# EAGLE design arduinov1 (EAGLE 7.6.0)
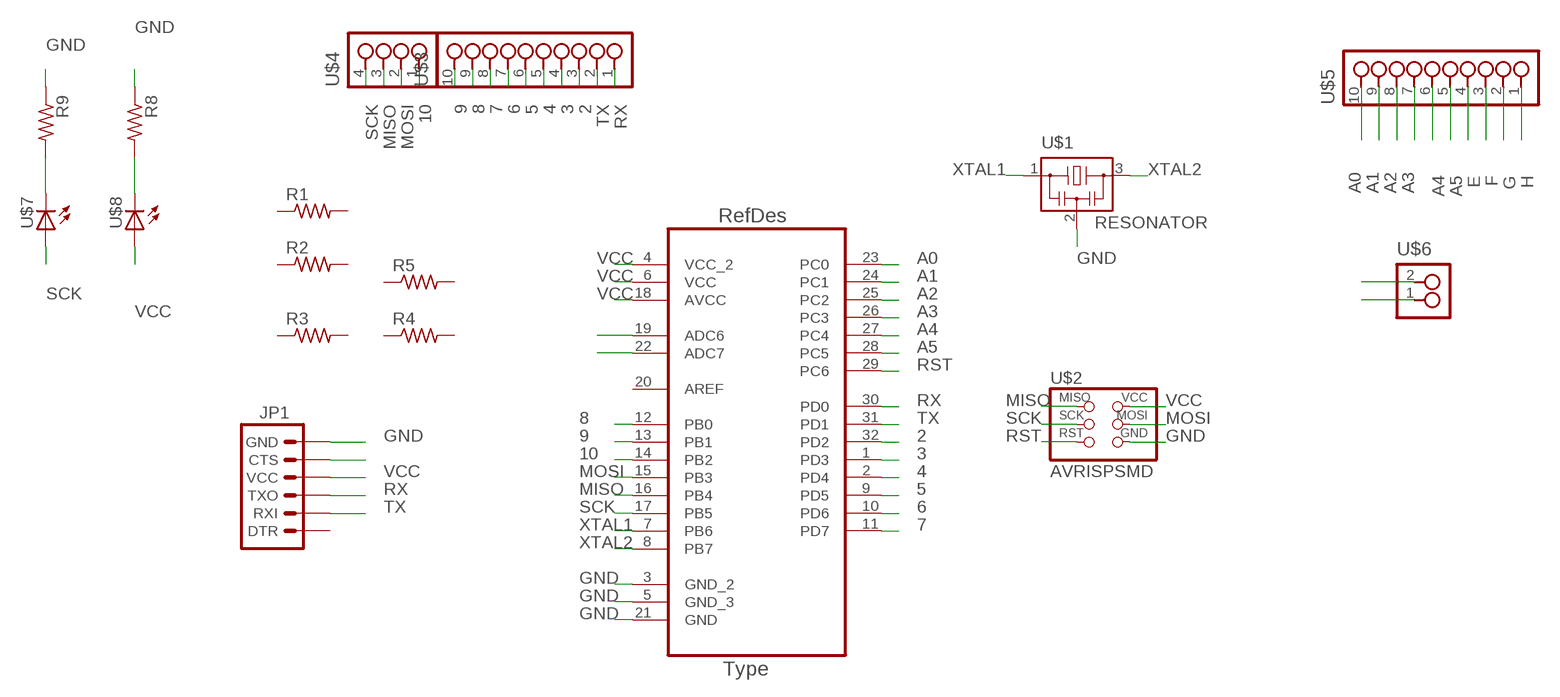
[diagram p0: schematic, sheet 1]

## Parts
JP1  ARDUINO_SERIAL_PROGRAMSMD  [1X06-SMD]
R1  RES-US1206FAB  [R1206FAB]
R2  RES-US1206FAB  [R1206FAB]
R3  RES-US1206FAB  [R1206FAB]
R4  RES-US1206FAB  [R1206FAB]
R5  RES-US1206FAB  [R1206FAB]
R8  RES-US1206FAB  [R1206FAB]
R9  RES-US1206FAB  [R1206FAB]
U1  ATMEGA328P-AU  [QFP80P900X900X120-32N]
U$1  RESONATOR  [EFOBM]
U$2  AVRISPSMD  [2X03SMD]
U$3  10_PIN_HEADERHEADER  [SMT_PINS_10]
U$4  4_PIN_HEADERHEADER  [SMT_PINS_4]
U$5  10_PIN_HEADERHEADER  [SMT_PINS_10]
U$6  2_PIN_HEADERHEADER  [SMT_PINS_2]
U$7  LED1206  [1206]
U$8  LED1206  [1206]

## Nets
2: U1.32(PD2) U$3.3
3: U1.1(PD3) U$3.4
4: U1.2(PD4) U$3.5
5: U1.9(PD5) U$3.6
6: U1.10(PD6) U$3.7
7: U1.11(PD7) U$3.8
8: U1.12(PB0) U$3.9
9: U1.13(PB1) U$3.10
10: U1.14(PB2) U$4.1
A0: U1.23(PC0) U$5.10
A1: U1.24(PC1) U$5.9
A2: U1.25(PC2) U$5.8
A3: U1.26(PC3) U$5.7
A4: U1.27(PC4) U$5.6
A5: U1.28(PC5) U$5.5
A6: U1.19(ADC6) U$6.1
A7: U1.22(ADC7) U$6.2
E: U$5.4
F: U$5.3
G: U$5.2
GND: JP1.6(GND) R8.1 R9.1 U1.3(GND_2) U1.5(GND_3) U1.21(GND) U$1.2 U$2.6(GND)
H: U$5.1
MISO: U1.16(PB4) U$2.1(MISO) U$4.3
MOSI: U1.15(PB3) U$2.4(MOSI) U$4.2
N$4: JP1.5(CTS)
N$7: R9.2 U$7.2(C)
N$8: R8.2 U$8.2(C)
RST: U1.29(PC6) U$2.5(RST)
RX: JP1.3(TXO) U1.30(PD0) U$3.1
SCK: U1.17(PB5) U$2.3(SCK) U$4.4 U$7.1(A)
TX: JP1.2(RXI) U1.31(PD1) U$3.2
VCC: JP1.4(VCC) U1.4(VCC_2) U1.6(VCC) U1.18(AVCC) U$2.2(VCC) U$8.1(A)
XTAL1: U1.7(PB6) U$1.1
XTAL2: U1.8(PB7) U$1.3
Unconnected: JP1.1(DTR) R1.1 R1.2 R2.1 R2.2 R3.1 R3.2 R4.1 R4.2 R5.1 R5.2 U1.20(AREF)

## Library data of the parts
JP1 = SparkFun-Connectors:ARDUINO_SERIAL_PROGRAM: FTDI connector footprints
R1-R5 R8 R9 = fab:RES-US: Resistor (US Symbol)
U1 = Atmel-ATMEGA328P-AU:ATMEGA328P-AU; DESCRIPTION: 8-bit Microcontroller with In-System Programmable Flash; MPN: ATMEGA328P-AU; OC_FARNELL: 1715486; OC_NEWARK: 14R4631; PACKAGE: TQFP-32; SUPPLIER: Atmel
U$1 = fab:RESONATOR
U$2 = fab:AVRISP
U$3 U$5 = FabLab:10_PIN_HEADER
U$4 = FabLab:4_PIN_HEADER: 4 SMT pin pads
U$6 = FabLab:2_PIN_HEADER: 2 SMT pin pads
U$7 U$8 = FabLab:LED

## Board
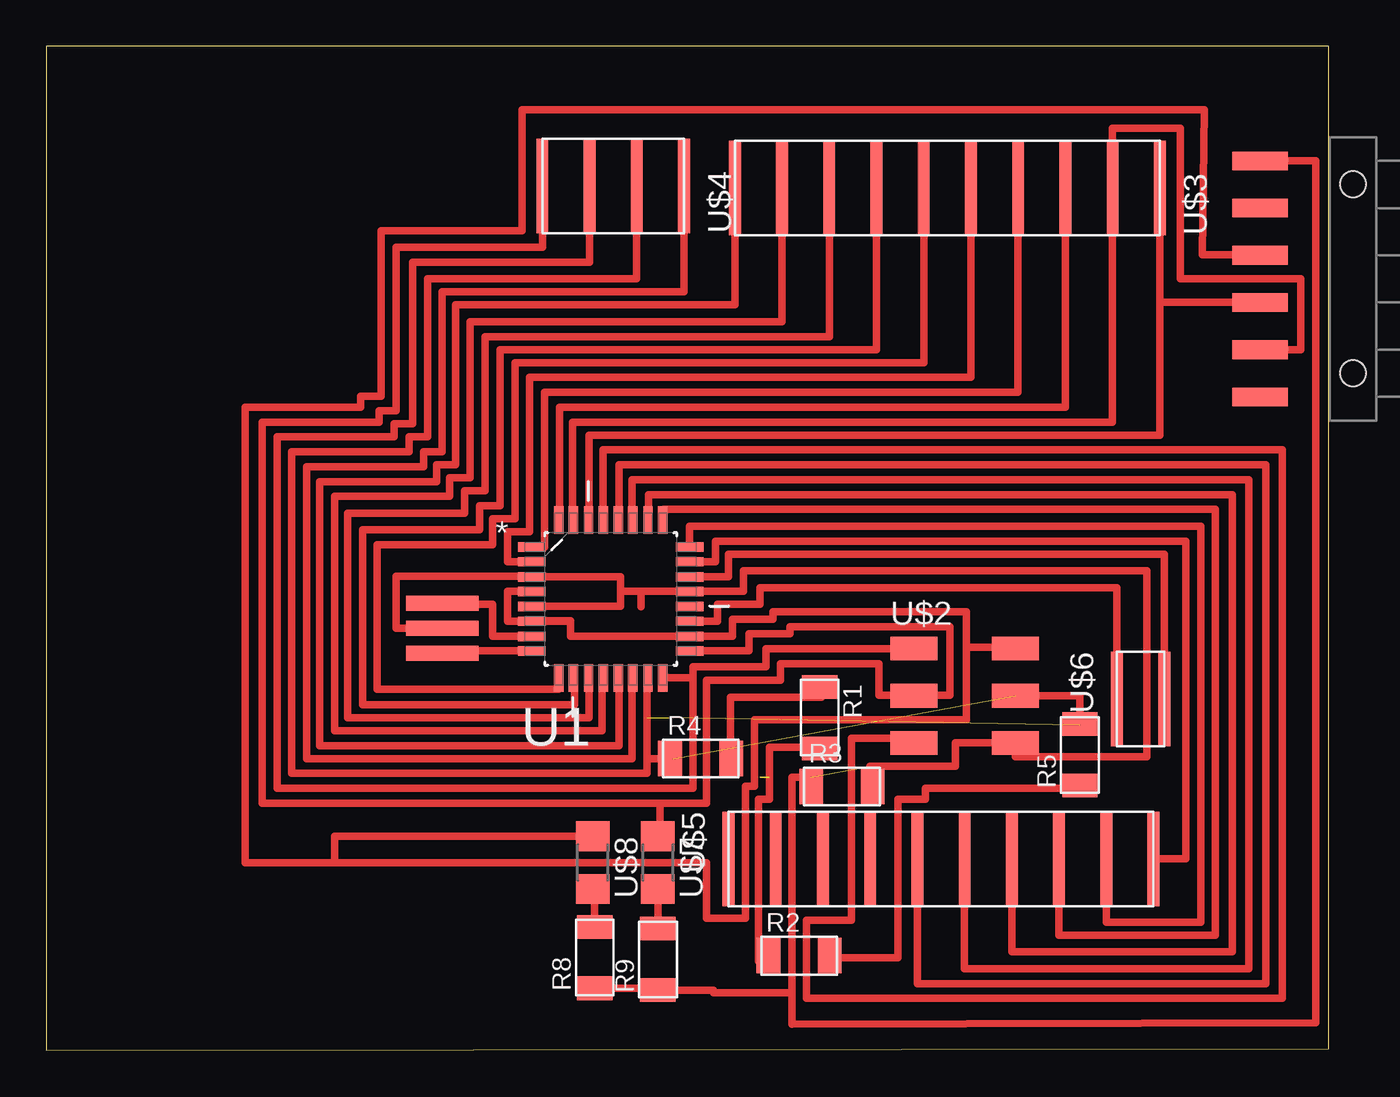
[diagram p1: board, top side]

Size 69 x 54 mm. Coordinates in mm from the lower left corner, seen from the top.
Outline: 0,0 69,0.1 69,54 0,54 0,0
Copper layers (1*16): Top 0.035mm / dielectric 1.5mm / Bottom 0.035mm
Design rules "default": minimum track width 10mil, minimum drill 24mil, track to track 8mil, track to pad 8mil, pad to pad 8mil, via to via 8mil, smd to smd 8mil, copper to edge 40mil, drill to drill 8mil, minimum pad ring 10mil, minimum via ring 8mil, stop-mask expansion 4mil, vias tented up to drill 0mil, thermal gap 10mil

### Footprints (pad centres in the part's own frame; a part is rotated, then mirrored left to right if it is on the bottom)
1X06-SMD = smd 1 x 3: 1 -6.35,5; 2 -3.81,5; 3 -1.27,5; 4 1.27,5; 5 3.81,5; 6 6.35,5 | hole 1.4: -5.08,0; 5.08,0
R1206FAB = smd 1.27 x 1.905: 1 -1.651,0; 2 1.651,0
QFP80P900X900X120-32N = smd 1.473 x 0.508: 1 -4.242,2.794; 2 -4.242,2.007; 3 -4.242,1.194; 4 -4.242,0.406; 5 -4.242,-0.406; 6 -4.242,-1.194; 7 -4.242,-2.007; 8 -4.242,-2.794; 17 4.242,-2.794; 18 4.242,-2.007; 19 4.242,-1.194; 20 4.242,-0.406; 21 4.242,0.406; 22 4.242,1.194; 23 4.242,2.007; 24 4.242,2.794 | smd 0.508 x 1.473: 9 -2.794,-4.242; 10 -2.007,-4.242; 11 -1.194,-4.242; 12 -0.406,-4.242; 13 0.406,-4.242; 14 1.194,-4.242; 15 2.007,-4.242; 16 2.794,-4.242; 25 2.794,4.242; 26 2.007,4.242; 27 1.194,4.242; 28 0.406,4.242; 29 -0.406,4.242; 30 -1.194,4.242; 31 -2.007,4.242; 32 -2.794,4.242
EFOBM = smd 0.8 x 3.9: 1 -1.35,0; 2 0,0; 3 1.35,0
2X03SMD = smd 2.54 x 1.27: 1 -2.54,2.54; 2 2.92,2.54; 3 -2.54,0; 4 2.92,0; 5 -2.54,-2.54; 6 2.92,-2.54
SMT_PINS_10 = smd 5.08 x 0.635: 1 0,0; 2 0,2.54; 3 0,5.08; 4 0,7.62; 5 0,10.16; 6 0,12.7; 7 0,15.24; 8 0,17.78; 9 0,20.32; 10 0,22.86
SMT_PINS_4 = smd 5.08 x 0.635: 1 0,0; 2 0,2.54; 3 0,5.08; 4 0,7.62
SMT_PINS_2 = smd 5.08 x 0.635: 1 0,0; 2 0,2.54
1206 = smd 1.6 x 1.803: 1 -1.422,0; 2 1.422,0

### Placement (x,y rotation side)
JP1  70.3,41.5 90 top
R1  41.6,17.9 270 top
R2  40.5,5.1 0 top
R3  42.8,14.2 0 top
R4  35.2,15.7 0 top
R5  55.6,15.9 90 top
R8  29.5,5 90 top
R9  32.9,4.9 90 top
U1  30.36,24.28 0 top
U$1  21.3,22.71 270 top
U$2  49.22,19.08 0 top
U$3  59.9,46.4 90 top
U$4  34.3,46.5 90 top
U$5  36.7,10.3 270 top
U$6  57.6,18.9 270 top
U$7  32.9,10.1 270 top
U$8  29.4,10.1 270 top

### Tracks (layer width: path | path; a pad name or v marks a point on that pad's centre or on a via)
2
  Top 0.406: U1.32 27.6,28.52 27.6,34.6 54.82,34.6 U$3.3
3
  Top 0.406: U1.1 26.8,27.07 26.8,35.4 52.28,35.4 U$3.4
4
  Top 0.406: U1.2 24.8,26.29 24.8,27.9 26,27.9 26,36.2 49.74,36.2 U$3.5
5
  Top 0.406: U$3.6 47.2,37 25.2,37 25.2,28.6 24,28.6 24,27.2 17.8,27.2 17.8,19.44 27.57,19.44 U1.9
6
  Top 0.406: U1.10 28.4,20.04 28.4,18.6 17,18.6 17,28 23.3,28 23.3,29.3 24.4,29.3 24.4,37.7 44.66,37.7 U$3.7
7
  Top 0.406: U1.11 29.2,20.04 29.2,17.9 16.2,17.9 16.2,28.9 22.5,28.9 22.5,30.1 23.6,30.1 23.6,38.4 42.12,38.4 U$3.8
8
  Top 0.406: U1.12 29.9,20.04 29.9,17.2 15.5,17.2 15.5,29.8 21.7,29.8 21.7,30.8 22.8,30.8 22.8,39.2 39.58,39.2 U$3.9
9
  Top 0.406: U1.13 30.8,20.04 30.8,16.4 14.7,16.4 14.7,30.6 21,30.6 21,31.5 22,31.5 22,40.1 37.04,40.1 U$3.10
10
  Top 0.406: U1.14 31.5,20.04 31.5,15.7 14,15.7 14,31.4 20.3,31.4 20.3,32.2 21.3,32.2 21.3,40.8 34.3,40.8 U$4.1
A0
  Top 0.406: U1.23 36,26.29 36,27.4 61.3,27.4 61.3,10.3 U$5.10
A1
  Top 0.406: U1.24 34.6,28.2 62.1,28.2 62.1,6.9 57.02,6.9 U$5.9
A2
  Top 0.406: U$5.8 54.48,6.2 62.9,6.2 62.9,29.1 33.2,29.1 33.2,28.52 U1.25
A3
  Top 0.406: U1.26 32.4,28.52 32.4,29.9 63.8,29.9 63.8,5.3 51.94,5.3 U$5.7
A4
  Top 0.406: U1.27 31.5,28.52 31.5,30.7 64.7,30.7 64.7,4.4 49.4,4.4 U$5.6
A5
  Top 0.406: U1.28 30.8,28.52 30.8,31.5 65.6,31.5 65.6,3.6 46.86,3.6 U$5.5
A6
  Top 0.406: U$6.1 57.6,24.9 38.4,24.9 38.4,24 36.1,24 36.1,23.09 U1.19
A7
  Top 0.406: U1.22 36.7,25.47 36.7,26.7 60.14,26.7 U$6.2
GND  (1 unrouted)
  Top 0.406: 30.9,24.69 30.9,25.47 U1.3 26.12,25.5 18.8,25.5 18.8,22.71 U$1.2 | 30.9,24.69 30.9,23.9 26.12,23.9 U1.5 | 32,24.69 U1.21 37.5,24.69 37.5,25.8 59.2,25.8 59.2,15.8 52.14,15.8 U$2.6 48.9,16.54 48.9,15.3 44.3,15.3 | 32,24.69 30.9,24.69 | 32,23.87 32,24.69 | JP1.6 68.3,47.85 68.3,1.5 40.1,1.4 40.1,3 40.1,3.1 | 40.1,3.1 40.1,14.7 41.1,14.7 | R8.1 32.9,3.35 R9.1 35.9,3.25 35.9,3.1 40.1,3.1
MISO
  Top 0.406: 34.8,20.04 34.8,20.64 38.7,20.64 38.7,21.6 46.68,21.6 U$2.1 | 34.8,20.04 34.8,14.1 12.4,14.1 12.4,33 18.7,33 18.7,33.7 19.7,33.7 19.7,42.4 29.22,42.4 U$4.3 | U1.16 34.8,20.04
MOSI  (3 unrouted)
  Top 0.406: 32.3,15.7 32.3,14.9 13.2,14.9 13.2,32.2 19.5,32.2 19.5,33 20.5,33 20.5,41.5 31.76,41.5 U$4.2 | U1.15 32.3,20.04 32.3,15.7 | U$2.4 55.6,19.08 55.6,17.5 | 32.3,15.7 33.7,15.7
N$1
  Top 0.406: 55.7,14.1 47.3,14.1 47.3,13.5 45.8,13.5 45.8,5 42.3,5
N$2  (2 unrouted)
  Top 0.406: 38.8,4.8 38.3,4.8 38.3,13.5 38.9,13.5 38.9,14.7
N$3
  Top 0.406: 41.2,16.3 38.9,16.3 38.9,13.5 38.3,13.5 38.3,5.3 38.8,5.3 38.8,5.4
N$5
  Top 0.406: 41.7,19.6 41.7,19.1
N$6
  Top 0.406: 36.8,15.7 36.8,19 41.7,19 41.7,19.7
N$7
  Top 0.406: U$7.2 R9.2
N$8
  Top 0.406: U$8.2 29.5,8.68 R8.2
RST
  Top 0.406: U1.29 29.95,32.3 66.5,32.3 66.5,2.8 40.9,2.8 40.9,7 43.3,7 43.3,16.8 46.68,16.8 U$2.5
RX
  Top 0.406: U1.30 29.2,28.52 29.2,33.1 59.9,33.1 59.9,40.23 | U$3.1 59.9,40.5 59.9,40.23 | JP1.3 59.9,40.23
SCK
  Top 0.406: 46.68,19.1 48.6,19.1 48.6,22.8 40,22.8 40,22.4 37.8,22.4 37.8,21.49 U1.17 | 46.68,19.1 U$2.3 | 46.68,19.1 44.8,19.1 44.8,20.8 39.5,20.8 39.5,19.9 35.5,19.9 35.5,13.3 33,13.3 | 33,13.3 11.6,13.3 11.6,33.8 17.9,33.8 17.9,34.4 18.8,34.4 18.8,43.2 26.68,43.2 U$4.4 | U$7.1 33,11.52 33,13.3
TX
  Top 0.406: U1.31 28.3,28.52 28.3,33.8 57.36,33.8 U$3.2 57.36,49.6 61,49.6 61,41.5 67.5,41.5 67.5,37.69 JP1.2
VCC
  Top 0.406: 28.2,23.09 28.2,23.1 U1.6 | U1.6 24.8,23.09 24.8,24.7 U1.4 | 49.5,21.7 49.5,23.6 39.1,23.6 39.1,23.2 36.9,23.2 36.9,22.27 U1.18 28.2,22.27 28.2,23.09 | 49.5,21.7 52.14,21.7 U$2.2 | U1.6 28.2,23.09 | 49.5,21.7 49.5,17.8 38.1,17.8 38.1,14.2 37.6,14.2 37.6,7.1 35.5,7.1 35.5,10.1 15.5,10.1 | 15.5,10.1 10.7,10.1 10.7,34.6 16.9,34.6 16.9,35.2 18,35.2 18,44.1 25.6,44.1 25.6,50.6 62.3,50.6 62.2,42.8 65.3,42.8 JP1.4 | U$8.1 15.5,11.52 15.5,10.1
XTAL1
  Top 0.406: U1.7 24,22.27 24,24 21.3,24 U$1.1
XTAL2
  Top 0.406: U1.8 21.7,21.49 U$1.3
